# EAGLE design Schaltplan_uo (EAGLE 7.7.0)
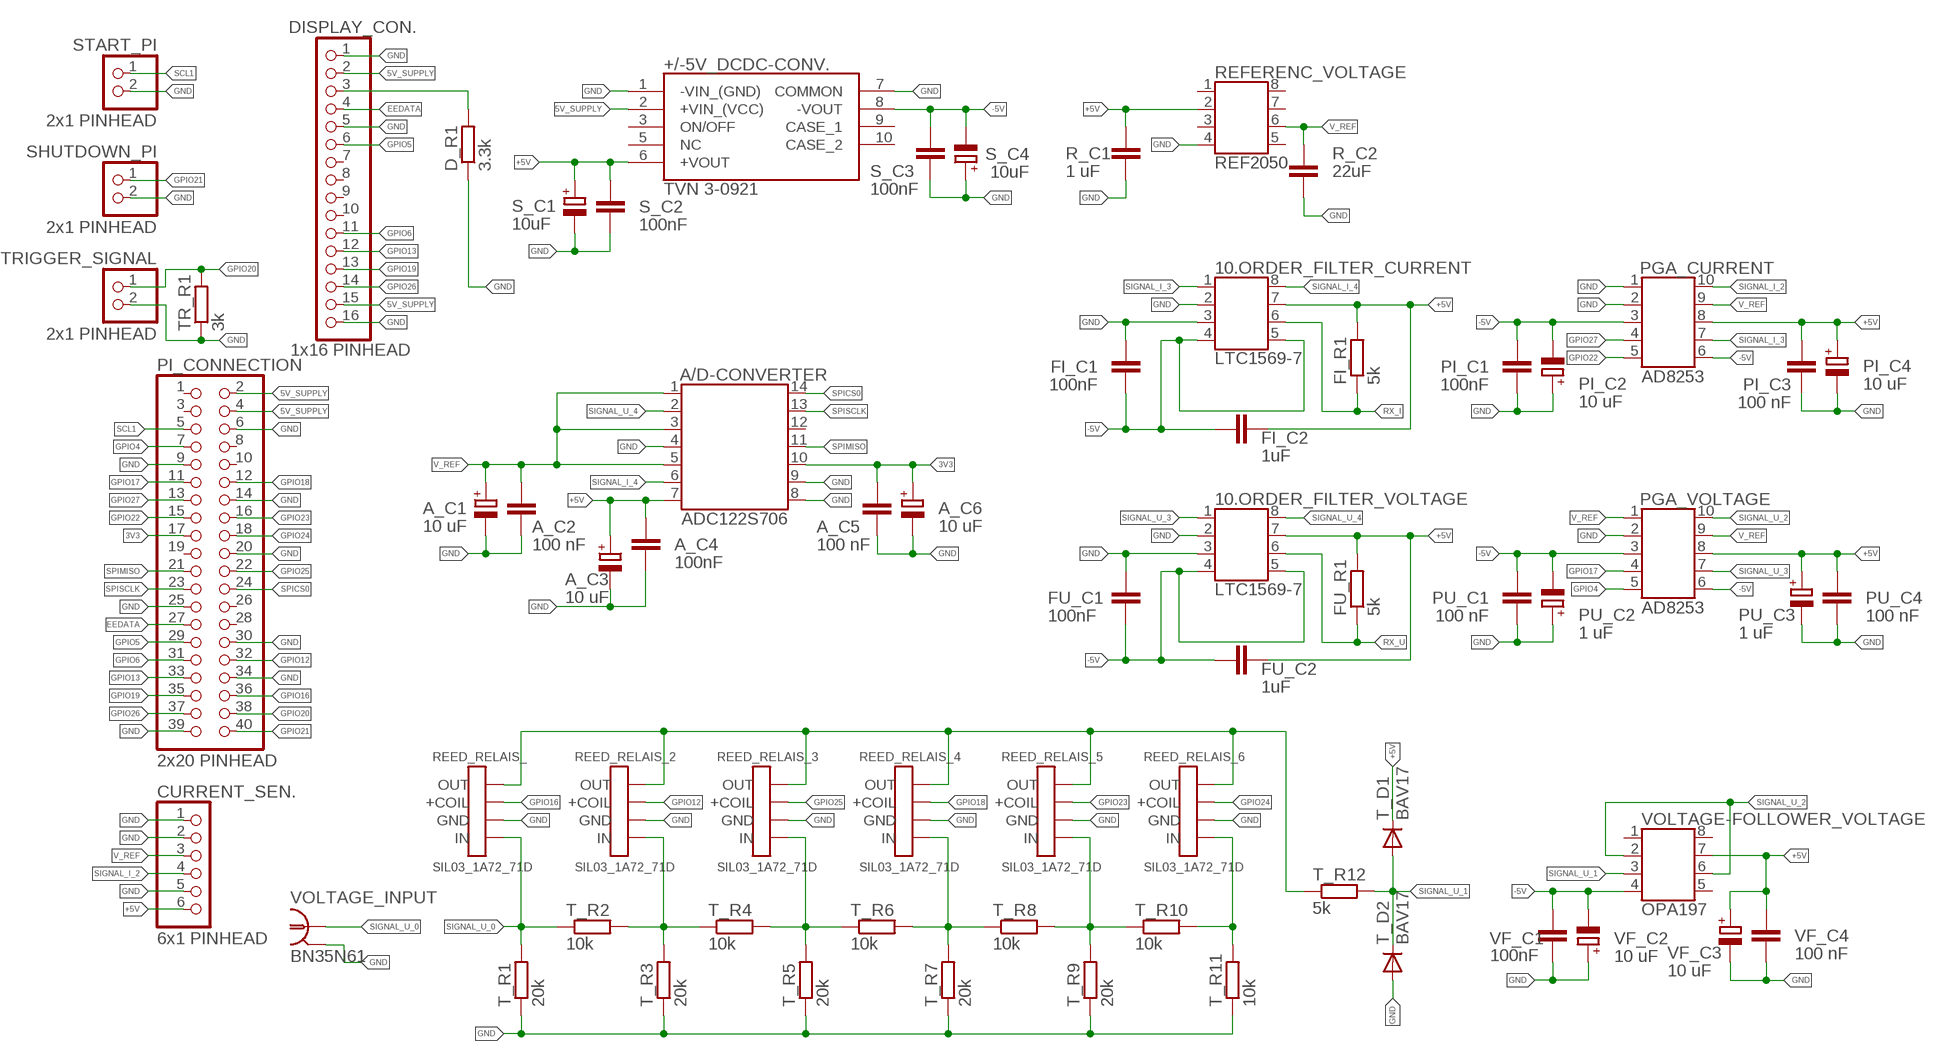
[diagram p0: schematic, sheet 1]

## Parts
10.ORDER_FILTER_CURRENT  LTC1569-7  SSOP8_TO_DIP8  [SSOP8_TO_DIP8]
10.ORDER_FILTER_VOLTAGE  LTC1569-7  SSOP8_TO_DIP8  [SSOP8_TO_DIP8]
+/-5V_DCDC-CONV.  TVN 3-0921  TVN_3-1223  [TVN32419]
A/D-CONVERTER  ADC122S706  SSOP14_TO_DIP14-6  [SSOP14_TO_DIP14-6]
A_C1  10 uF  CPOL-EUE2.5-6  [E2,5-6]
A_C2  100 nF  C-EU025-030X050  [C025-030X050]
A_C3  10 uF  CPOL-EUE2.5-6  [E2,5-6]
A_C4  100nF  C-EU025-030X050  [C025-030X050]
A_C5  100 nF  C-EU025-030X050  [C025-030X050]
A_C6  10 uF  CPOL-EUE2.5-6  [E2,5-6]
CURRENT_SEN.  6x1 PINHEAD  PINHD-1X6  [1X06]
D_R1  3.3k  R-EU_0207/10  [0207/10]
DISPLAY_CON.  1x16 PINHEAD  PINHD-1X16  [1X16]
FI_C1  100nF  C-EU025-030X050  [C025-030X050]
FI_C2  1uF  C-EU025-030X050  [C025-030X050]
FI_R1  5k  R-EU_0207/10  [0207/10]
FU_C1  100nF  C-EU025-030X050  [C025-030X050]
FU_C2  1uF  C-EU025-030X050  [C025-030X050]
FU_R1  5k  R-EU_0207/10  [0207/10]
PGA_CURRENT  AD8253  SSOP10_TO_DIP10  [SSOP10_TO_DIP10]
PGA_VOLTAGE  AD8253  SSOP10_TO_DIP10  [SSOP10_TO_DIP10]
PI_C1  100nF  C-EU025-030X050  [C025-030X050]
PI_C2  10 uF  CPOL-EUE2.5-6  [E2,5-6]
PI_C3  100 nF  C-EU025-030X050  [C025-030X050]
PI_C4  10 uF  CPOL-EUE2.5-6  [E2,5-6]
PI_CONNECTION  2x20 PINHEAD  PINHD-2X20  [2X20]
PU_C1  100 nF  C-EU025-030X050  [C025-030X050]
PU_C2  1 uF  CPOL-EUE2.5-6  [E2,5-6]
PU_C3  1 uF  CPOL-EUE2.5-6  [E2,5-6]
PU_C4  100 nF  C-EU025-030X050  [C025-030X050]
R_C1  1 uF  C-EU025-030X050  [C025-030X050]
R_C2  22uF  C-EU025-030X050  [C025-030X050]
REED_RELAIS_  SIL03_1A72_71D  REED_REALIS_SIL03_1A72_71D  [REED_RELAIS_SIL03_1A72_71D]
REED_RELAIS_2  SIL03_1A72_71D  REED_REALIS_SIL03_1A72_71D  [REED_RELAIS_SIL03_1A72_71D]
REED_RELAIS_3  SIL03_1A72_71D  REED_REALIS_SIL03_1A72_71D  [REED_RELAIS_SIL03_1A72_71D]
REED_RELAIS_4  SIL03_1A72_71D  REED_REALIS_SIL03_1A72_71D  [REED_RELAIS_SIL03_1A72_71D]
REED_RELAIS_5  SIL03_1A72_71D  REED_REALIS_SIL03_1A72_71D  [REED_RELAIS_SIL03_1A72_71D]
REED_RELAIS_6  SIL03_1A72_71D  REED_REALIS_SIL03_1A72_71D  [REED_RELAIS_SIL03_1A72_71D]
REFERENC_VOLTAGE  REF2050  SSOP8_TO_DIP8  [SSOP8_TO_DIP8]
S_C1  10uF  CPOL-EUE2.5-6  [E2,5-6]
S_C2  100nF  C-EU025-030X050  [C025-030X050]
S_C3  100nF  C-EU025-030X050  [C025-030X050]
S_C4  10uF  CPOL-EUE2.5-6  [E2,5-6]
SHUTDOWN_PI  2x1 PINHEAD  PINHD-1X2  [1X02]
START_PI  2x1 PINHEAD  PINHD-1X2  [1X02]
T_D1  BAV17  [DO35-10]
T_D2  BAV17  [DO35-10]
T_R1  20k  R-EU_0207/10  [0207/10]
T_R2  10k  R-EU_0207/10  [0207/10]
T_R3  20k  R-EU_0207/10  [0207/10]
T_R4  10k  R-EU_0207/10  [0207/10]
T_R5  20k  R-EU_0207/10  [0207/10]
T_R6  10k  R-EU_0207/10  [0207/10]
T_R7  20k  R-EU_0207/10  [0207/10]
T_R8  10k  R-EU_0207/10  [0207/10]
T_R9  20k  R-EU_0207/10  [0207/10]
T_R10  10k  R-EU_0207/10  [0207/10]
T_R11  10k  R-EU_0207/10  [0207/10]
T_R12  5k  R-EU_0207/10  [0207/10]
TR_R1  3k  R-EU_0207/10  [0207/10]
TRIGGER_SIGNAL  2x1 PINHEAD  PINHD-1X2  [1X02]
VF_C1  100nF  C-EU025-030X050  [C025-030X050]
VF_C2  10 uF  CPOL-EUE2.5-6  [E2,5-6]
VF_C3  10 uF  CPOL-EUE2.5-6  [E2,5-6]
VF_C4  100 nF  C-EU025-030X050  [C025-030X050]
VOLTAGE-FOLLOWER_VOLTAGE  OPA197  SSOP8_TO_DIP8  [SSOP8_TO_DIP8]
VOLTAGE_INPUT  BN35N61  [B35N61]

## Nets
3V3: A/D-CONVERTER.10 A_C5.1 A_C6.+ PI_CONNECTION.17
5V_SUPPLY: +/-5V_DCDC-CONV..2(+VIN_(VCC)) DISPLAY_CON..2 DISPLAY_CON..15 PI_CONNECTION.2 PI_CONNECTION.4
+5V: 10.ORDER_FILTER_CURRENT.7 10.ORDER_FILTER_VOLTAGE.7 +/-5V_DCDC-CONV..6(+VOUT) A/D-CONVERTER.7 A_C3.+ A_C4.1 CURRENT_SEN..6 FI_C2.2 FI_R1.2 FU_C2.1 FU_R1.2 PGA_CURRENT.8 PGA_VOLTAGE.8 PI_C3.1 PI_C4.+ PU_C3.+ PU_C4.1 R_C1.1 REFERENC_VOLTAGE.2 S_C1.+ S_C2.1 T_D1.C VF_C3.+ VF_C4.1 VOLTAGE-FOLLOWER_VOLTAGE.7
-5V: 10.ORDER_FILTER_CURRENT.4 10.ORDER_FILTER_CURRENT.5 10.ORDER_FILTER_VOLTAGE.4 10.ORDER_FILTER_VOLTAGE.5 +/-5V_DCDC-CONV..8(-VOUT) FI_C1.1 FI_C2.1 FU_C1.1 FU_C2.2 PGA_CURRENT.3 PGA_CURRENT.6 PGA_VOLTAGE.3 PGA_VOLTAGE.6 PI_C1.1 PI_C2.- PU_C1.1 PU_C2.- S_C3.1 S_C4.- VF_C1.1 VF_C2.- VOLTAGE-FOLLOWER_VOLTAGE.4
EEDATA: DISPLAY_CON..4 PI_CONNECTION.27
GND: 10.ORDER_FILTER_CURRENT.2 10.ORDER_FILTER_CURRENT.3 10.ORDER_FILTER_VOLTAGE.2 10.ORDER_FILTER_VOLTAGE.3 +/-5V_DCDC-CONV..1(-VIN_(GND)) +/-5V_DCDC-CONV..7(COMMON) A/D-CONVERTER.4 A/D-CONVERTER.8 A/D-CONVERTER.9 A_C1.- A_C2.2 A_C3.- A_C4.2 A_C5.2 A_C6.- CURRENT_SEN..1 CURRENT_SEN..2 CURRENT_SEN..5 D_R1.1 DISPLAY_CON..1 DISPLAY_CON..5 DISPLAY_CON..16 FI_C1.2 FU_C1.2 PGA_CURRENT.1 PGA_CURRENT.2 PGA_VOLTAGE.2 PI_C1.2 PI_C2.+ PI_C3.2 PI_C4.- PI_CONNECTION.6 PI_CONNECTION.9 PI_CONNECTION.14 PI_CONNECTION.20 PI_CONNECTION.25 PI_CONNECTION.30 PI_CONNECTION.34 PI_CONNECTION.39 PU_C1.2 PU_C2.+ PU_C3.- PU_C4.2 R_C1.2 R_C2.2 REED_RELAIS_2.P$3(GND) REED_RELAIS_3.P$3(GND) REED_RELAIS_4.P$3(GND) REED_RELAIS_5.P$3(GND) REED_RELAIS_6.P$3(GND) REED_RELAIS_.P$3(GND) REFERENC_VOLTAGE.4 S_C1.- S_C2.2 S_C3.2 S_C4.+ SHUTDOWN_PI.2 START_PI.2 T_D2.A T_R1.1 T_R3.1 T_R5.1 T_R7.1 T_R9.1 T_R11.1 TR_R1.1 TRIGGER_SIGNAL.2 VF_C1.2 VF_C2.+ VF_C3.- VF_C4.2 VOLTAGE_INPUT.2 VOLTAGE_INPUT.3 VOLTAGE_INPUT.4 VOLTAGE_INPUT.5
GPIO4: PGA_VOLTAGE.5 PI_CONNECTION.7
GPIO5: DISPLAY_CON..6 PI_CONNECTION.29
GPIO6: DISPLAY_CON..11 PI_CONNECTION.31
GPIO12: PI_CONNECTION.32 REED_RELAIS_2.P$2(+COIL)
GPIO13: DISPLAY_CON..12 PI_CONNECTION.33
GPIO16: PI_CONNECTION.36 REED_RELAIS_.P$2(+COIL)
GPIO17: PGA_VOLTAGE.4 PI_CONNECTION.11
GPIO18: PI_CONNECTION.12 REED_RELAIS_4.P$2(+COIL)
GPIO19: DISPLAY_CON..13 PI_CONNECTION.35
GPIO20: PI_CONNECTION.38 TR_R1.2 TRIGGER_SIGNAL.1
GPIO21: PI_CONNECTION.40 SHUTDOWN_PI.1
GPIO22: PGA_CURRENT.5 PI_CONNECTION.15
GPIO23: PI_CONNECTION.16 REED_RELAIS_5.P$2(+COIL)
GPIO24: PI_CONNECTION.18 REED_RELAIS_6.P$2(+COIL)
GPIO25: PI_CONNECTION.22 REED_RELAIS_3.P$2(+COIL)
GPIO26: DISPLAY_CON..14 PI_CONNECTION.37
GPIO27: PGA_CURRENT.4 PI_CONNECTION.13
N$2: REED_RELAIS_2.P$1(OUT) REED_RELAIS_3.P$1(OUT) REED_RELAIS_4.P$1(OUT) REED_RELAIS_5.P$1(OUT) REED_RELAIS_6.P$1(OUT) REED_RELAIS_.P$1(OUT) T_R12.1
N$3: D_R1.2 DISPLAY_CON..3
N$42: REED_RELAIS_2.P$4(IN) T_R2.2 T_R3.2 T_R4.1
N$43: REED_RELAIS_3.P$4(IN) T_R4.2 T_R5.2 T_R6.1
N$44: REED_RELAIS_4.P$4(IN) T_R6.2 T_R7.2 T_R8.1
N$45: REED_RELAIS_5.P$4(IN) T_R8.2 T_R9.2 T_R10.1
N$46: REED_RELAIS_6.P$4(IN) T_R10.2 T_R11.2
RX_I: 10.ORDER_FILTER_CURRENT.6 FI_R1.1
RX_U: 10.ORDER_FILTER_VOLTAGE.6 FU_R1.1
SCL1: PI_CONNECTION.5 START_PI.1
SIGNAL_I_2: CURRENT_SEN..4 PGA_CURRENT.10
SIGNAL_I_3: 10.ORDER_FILTER_CURRENT.1 PGA_CURRENT.7
SIGNAL_I_4: 10.ORDER_FILTER_CURRENT.8 A/D-CONVERTER.6
SIGNAL_U_0: REED_RELAIS_.P$4(IN) T_R1.2 T_R2.1 VOLTAGE_INPUT.1
SIGNAL_U_1: T_D1.A T_D2.C T_R12.2 VOLTAGE-FOLLOWER_VOLTAGE.3
SIGNAL_U_2: PGA_VOLTAGE.10 VOLTAGE-FOLLOWER_VOLTAGE.2 VOLTAGE-FOLLOWER_VOLTAGE.6
SIGNAL_U_3: 10.ORDER_FILTER_VOLTAGE.1 PGA_VOLTAGE.7
SIGNAL_U_4: 10.ORDER_FILTER_VOLTAGE.8 A/D-CONVERTER.2
SPICS0: A/D-CONVERTER.14 PI_CONNECTION.24
SPIMISO: A/D-CONVERTER.11 PI_CONNECTION.21
SPISCLK: A/D-CONVERTER.13 PI_CONNECTION.23
V_REF: A/D-CONVERTER.1 A/D-CONVERTER.3 A/D-CONVERTER.5 A_C1.+ A_C2.1 CURRENT_SEN..3 PGA_CURRENT.9 PGA_VOLTAGE.1 PGA_VOLTAGE.9 R_C2.1 REFERENC_VOLTAGE.6
Unconnected: +/-5V_DCDC-CONV..3(ON/OFF) +/-5V_DCDC-CONV..5(NC) +/-5V_DCDC-CONV..9(CASE_1) +/-5V_DCDC-CONV..10(CASE_2) A/D-CONVERTER.12 DISPLAY_CON..7 DISPLAY_CON..8 DISPLAY_CON..9 DISPLAY_CON..10 PI_CONNECTION.1 PI_CONNECTION.3 PI_CONNECTION.8 PI_CONNECTION.10 PI_CONNECTION.19 PI_CONNECTION.26 PI_CONNECTION.28 REFERENC_VOLTAGE.1 REFERENC_VOLTAGE.3 REFERENC_VOLTAGE.5 REFERENC_VOLTAGE.7 REFERENC_VOLTAGE.8 VOLTAGE-FOLLOWER_VOLTAGE.1 VOLTAGE-FOLLOWER_VOLTAGE.5 VOLTAGE-FOLLOWER_VOLTAGE.8

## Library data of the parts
10.ORDER_FILTER_CURRENT 10.ORDER_FILTER_VOLTAGE REFERENC_VOLTAGE VOLTAGE-FOLLOWER_VOLTAGE = OWN_Library:SSOP8_TO_DIP8
+/-5V_DCDC-CONV. = TVN_3-1223:TVN_3-1223: Isolated DC/DC Converters 3W 9-18Vin SIP-8 +/-15Vout +/-100mA Source: Datasheet; ALLIED_NUMBER: 71099550; ALLIED_PRICE-STOCK: https://www.alliedelec.com/traco-power-tvn-3-1223/71099550/; DESCRIPTION: Isolated DC/DC Converters 3W 9-18Vin SIP-8 +/-15Vout +/-100mA; HEIGHT: 11mm; MANUFACTURER_NAME: Traco Power; MANUFACTURER_PART_NUMBER: TVN 3-1223; MOUSER_PART_NUMBER: 495-TVN3-1223; MOUSER_PRICE-STOCK: https://www.mouser.com/Search/Refine.aspx?Keyword=495-TVN3-1223; RS_PART_NUMBER: 1466094; RS_PRICE-STOCK: https://uk.rs-online.com/web/p/products/1466094
A/D-CONVERTER = OWN_Library:SSOP14_TO_DIP14-6: SSOP14 SMD to DIP14-6 ADAPTER
A_C1 A_C3 A_C6 PI_C2 PI_C4 PU_C2 PU_C3 S_C1 S_C4 VF_C2 VF_C3 = rcl:CPOL-EU: POLARIZED CAPACITOR, European symbol
A_C2 A_C4 A_C5 FI_C1 FI_C2 FU_C1 FU_C2 PI_C1 PI_C3 PU_C1 PU_C4 R_C1 R_C2 S_C2 S_C3 VF_C1 VF_C4 = rcl:C-EU: CAPACITOR, European symbol
CURRENT_SEN. = pinhead:PINHD-1X6: PIN HEADER
D_R1 FI_R1 FU_R1 T_R1-T_R12 TR_R1 = rcl:R-EU_: RESISTOR, European symbol
DISPLAY_CON. = pinhead:PINHD-1X16: PIN HEADER
PGA_CURRENT PGA_VOLTAGE = OWN_Library:SSOP10_TO_DIP10
PI_CONNECTION = pinhead:PINHD-2X20: PIN HEADER
REED_RELAIS_ REED_RELAIS_2-REED_RELAIS_6 = OWN_Library:REED_REALIS_SIL03_1A72_71D
SHUTDOWN_PI START_PI TRIGGER_SIGNAL = pinhead:PINHD-1X2: PIN HEADER
T_D1 T_D2 = diode:BAV17: DIODE
VOLTAGE_INPUT = con-coax:BN35N61: BNC CONNECTOR; OC_FARNELL: unknown; OC_NEWARK: unknown

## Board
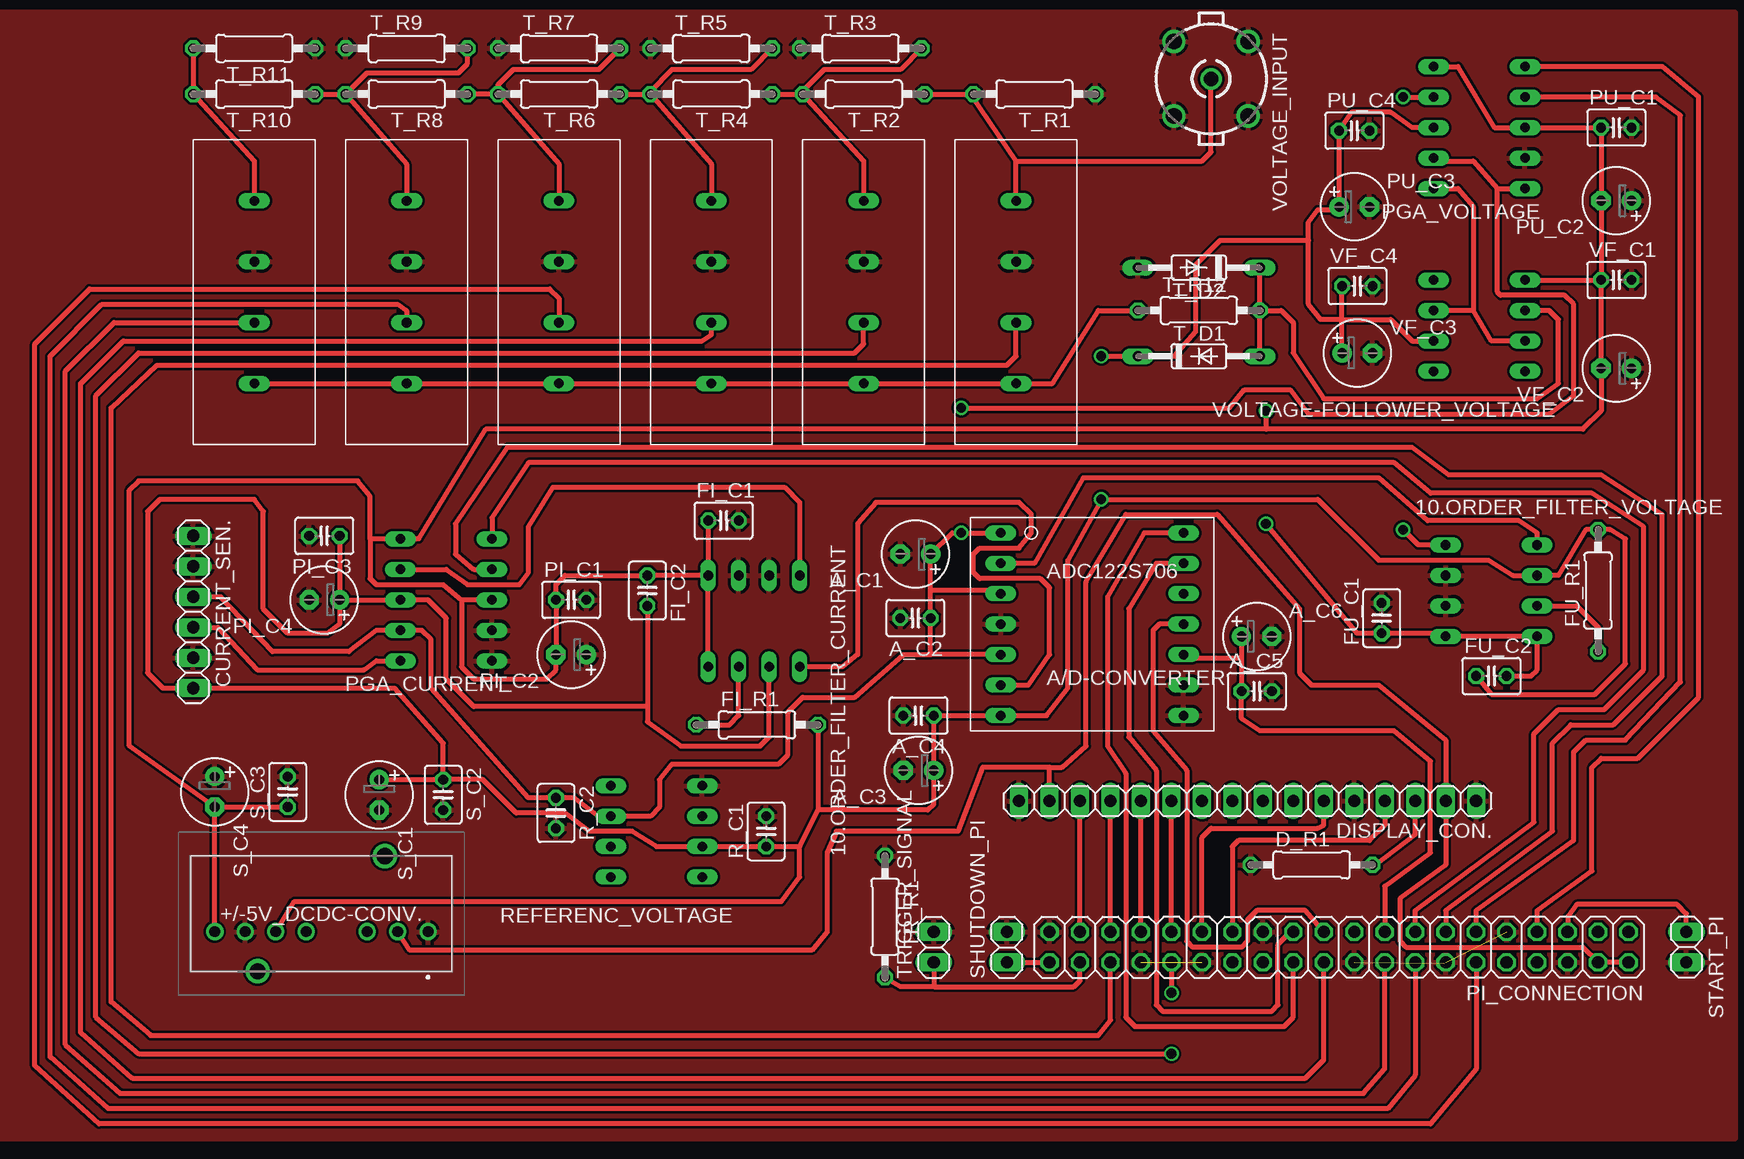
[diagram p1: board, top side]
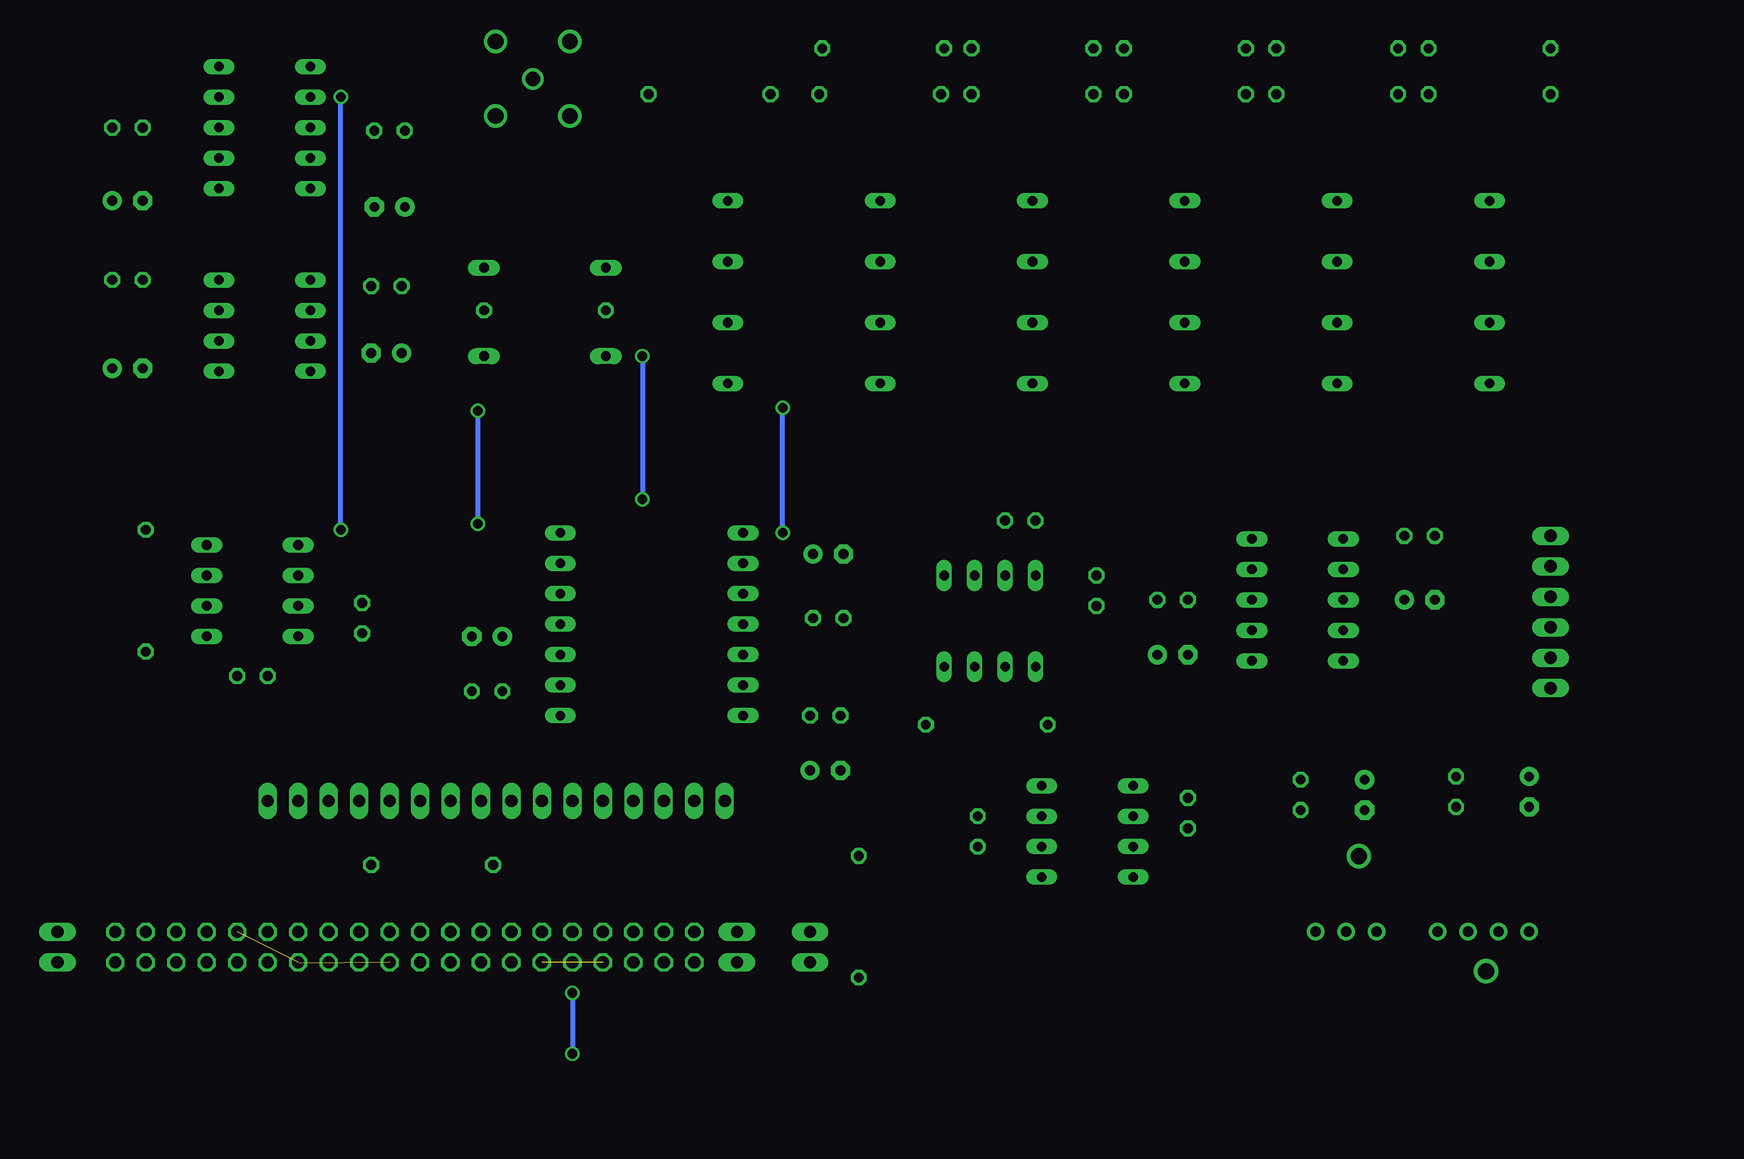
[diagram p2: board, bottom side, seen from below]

No outline drawn. Coordinates in mm, seen from the top.
Copper layers (1*16): Top 0.035mm / dielectric 1.5mm / Bottom 0.035mm
Design rules "default": minimum track width 10mil, minimum drill 24mil, track to track 8mil, track to pad 8mil, pad to pad 8mil, via to via 8mil, smd to smd 8mil, copper to edge 40mil, drill to drill 8mil, minimum pad ring 10mil, minimum via ring 8mil, stop-mask expansion 4mil, vias tented up to drill 0mil, thermal gap 10mil

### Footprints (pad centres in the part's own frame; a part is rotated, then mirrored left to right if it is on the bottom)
SSOP8_TO_DIP8 = drill 0.8 long: 1 -5.08,2.54; 2 -5.08,0; 3 -5.08,-2.54; 4 -5.08,-5.08; 5 2.54,-5.08; 6 2.54,-2.54; 7 2.54,0; 8 2.54,2.54
TVN32419 = drill 0.89 pad 1.446: 1 -8.9,1.5; 2 -6.36,1.5; 3 -3.82,1.5; 5 1.26,1.5; 6 3.8,1.5; 7 6.34,1.5; 8 8.88,1.5 | drill 1.35 pad 2.025: 9 -5.3,-4.8; 10 5.3,4.8
SSOP14_TO_DIP14-6 = drill 0.8 long: 1 -7.62,7.62; 2 -7.62,5.08; 3 -7.62,2.54; 4 -7.62,0; 5 -7.62,-2.54; 6 -7.62,-5.08; 7 -7.62,-7.62; 8 7.62,-7.62; 9 7.62,-5.08; 10 7.62,-2.54; 11 7.62,0; 12 7.62,2.54; 13 7.62,5.08; 14 7.62,7.62
E2,5-6 = drill 0.813 pad 1.6: + -1.27,0 | drill 0.813 pad 1.6 octagon: - 1.27,0
C025-030X050 = drill 0.813 octagon: 1 -1.27,0; 2 1.27,0
1X06 = drill 1.016 long: 1 -6.35,0; 2 -3.81,0; 3 -1.27,0; 4 1.27,0; 5 3.81,0; 6 6.35,0
0207/10 = drill 0.813 octagon: 1 -5.08,0; 2 5.08,0
1X16 = drill 1.016 long: 1 -19.05,0; 2 -16.51,0; 3 -13.97,0; 4 -11.43,0; 5 -8.89,0; 6 -6.35,0; 7 -3.81,0; 8 -1.27,0; 9 1.27,0; 10 3.81,0; 11 6.35,0; 12 8.89,0; 13 11.43,0; 14 13.97,0; 15 16.51,0; 16 19.05,0
SSOP10_TO_DIP10 = drill 0.8 long: 1 -2.54,2.54; 2 -2.54,0; 3 -2.54,-2.54; 4 -2.54,-5.08; 5 -2.54,-7.62; 6 5.08,-7.62; 7 5.08,-5.08; 8 5.08,-2.54; 9 5.08,0; 10 5.08,2.54
2X20 = drill 1.016 octagon: 1 -24.13,-1.27; 2 -24.13,1.27; 3 -21.59,-1.27; 4 -21.59,1.27; 5 -19.05,-1.27; 6 -19.05,1.27; 7 -16.51,-1.27; 8 -16.51,1.27; 9 -13.97,-1.27; 10 -13.97,1.27; 11 -11.43,-1.27; 12 -11.43,1.27; 13 -8.89,-1.27; 14 -8.89,1.27; 15 -6.35,-1.27; 16 -6.35,1.27; 17 -3.81,-1.27; 18 -3.81,1.27; 19 -1.27,-1.27; 20 -1.27,1.27; 21 1.27,-1.27; 22 1.27,1.27; 23 3.81,-1.27; 24 3.81,1.27; 25 6.35,-1.27; 26 6.35,1.27; 27 8.89,-1.27; 28 8.89,1.27; 29 11.43,-1.27; 30 11.43,1.27; 31 13.97,-1.27; 32 13.97,1.27; 33 16.51,-1.27; 34 16.51,1.27; 35 19.05,-1.27; 36 19.05,1.27; 37 21.59,-1.27; 38 21.59,1.27; 39 24.13,-1.27; 40 24.13,1.27
REED_RELAIS_SIL03_1A72_71D = drill 0.8 long: P$1 0,0; P$2 0,-5.08; P$3 0,-10.16; P$4 0,-15.24
1X02 = drill 1.016 long: 1 -1.27,0; 2 1.27,0
DO35-10 = drill 0.813 long: A 5.08,0; C -5.08,0
B35N61 = drill 1.2: 1 0,0 | drill 1.3: 2 3.099,3.099; 3 -3.099,3.099; 4 -3.099,-3.099; 5 3.099,-3.099

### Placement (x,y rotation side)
10.ORDER_FILTER_CURRENT  64.26,41.91 270 top
10.ORDER_FILTER_VOLTAGE  125.73,46.99 0 top
+/-5V_DCDC-CONV.  26.92,18.8 180 top
A/D-CONVERTER  91.19,42.93 0 top
A_C1  76.45,48.77 180 top
A_C2  76.45,43.43 180 top
A_C3  76.71,30.73 180 top
A_C4  76.71,35.31 180 top
A_C5  104.9,37.34 0 top
A_C6  104.9,41.91 0 top
CURRENT_SEN.  16.26,43.94 270 top
D_R1  109.47,22.86 0 top
DISPLAY_CON.  104.14,28.19 180 top
FI_C1  60.45,51.56 0 top
FI_C2  54.1,45.72 270 top
FI_R1  63.25,34.54 0 top
FU_C1  115.32,43.43 90 top
FU_C2  124.46,38.61 0 top
FU_R1  133.35,45.72 90 top
PGA_CURRENT  38.61,42.42 180 top
PGA_VOLTAGE  124.71,81.79 180 top
PI_C1  47.75,44.96 0 top
PI_C2  47.75,40.39 180 top
PI_C3  27.18,50.29 180 top
PI_C4  27.18,44.96 180 top
PI_CONNECTION  111.76,16 180 top
PU_C1  134.87,84.33 0 top
PU_C2  134.87,78.23 180 top
PU_C3  113.03,77.72 0 top
PU_C4  113.03,84.07 0 top
R_C1  64.01,25.65 90 top
R_C2  46.48,27.18 270 top
REED_RELAIS_  84.84,62.99 180 top
REED_RELAIS_2  72.14,62.99 180 top
REED_RELAIS_3  59.44,62.99 180 top
REED_RELAIS_4  46.74,62.99 180 top
REED_RELAIS_5  34.04,62.99 180 top
REED_RELAIS_6  21.34,62.99 180 top
REFERENC_VOLTAGE  53.59,24.38 180 top
S_C1  31.75,28.7 270 top
S_C2  37.08,28.7 270 top
S_C3  24.13,28.96 90 top
S_C4  18.03,28.96 270 top
SHUTDOWN_PI  84.07,16 90 top
START_PI  140.72,16 270 top
T_D1  100.08,65.28 0 top
T_D2  100.08,72.64 180 top
T_R1  86.36,87.12 180 top
T_R2  72.14,87.12 180 top
T_R3  71.88,90.93 0 top
T_R4  59.44,87.12 180 top
T_R5  59.44,90.93 0 top
T_R6  46.74,87.12 180 top
T_R7  46.74,90.93 0 top
T_R8  34.04,87.12 180 top
T_R9  34.04,90.93 0 top
T_R10  21.34,87.12 180 top
T_R11  21.34,90.93 180 top
T_R12  100.08,69.09 0 top
TR_R1  73.91,18.54 270 top
TRIGGER_SIGNAL  77.98,16 90 top
VF_C1  134.87,71.63 0 top
VF_C2  134.87,64.26 180 top
VF_C3  113.28,65.53 0 top
VF_C4  113.28,71.12 0 top
VOLTAGE-FOLLOWER_VOLTAGE  122.17,66.55 180 top
VOLTAGE_INPUT  101.09,88.39 270 top

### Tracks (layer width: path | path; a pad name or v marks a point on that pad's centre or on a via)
3V3
  Top 0.406: PI_CONNECTION.17 115.57,21.08 119.38,23.88 119.38,31.5 116.33,34.04 105.16,34.04 103.63,35.05 A_C5.1 103.63,40.13 | A_C6.+ 103.63,40.13 | A/D-CONVERTER.10 99.06,40.13 103.63,40.13
5V_SUPPLY
  Top 0.406: 87.63,30.99 82.04,30.99 80.01,25.65 69.85,25.65 69.09,23.88 69.09,17.27 67.82,15.75 34.29,15.75 33.3,17.3 +/-5V_DCDC-CONV..2 | PI_CONNECTION.2 PI_CONNECTION.4 132.08,16 117.35,16 116.84,16.51 116.84,20.07 120.65,22.86 DISPLAY_CON..2 120.65,33.27 115.06,37.85 109.47,37.85 108.46,38.86 108.46,44.2 101.6,52.07 93.98,52.07 90.68,46.48 90.68,32.77 88.65,30.99 87.63,30.99 | DISPLAY_CON..15 87.63,30.99
+5V  (via drill 0.8)
  Top 0.406: FU_C2.1 124.46,37.08 133.1,37.08 135.64,39.62 135.64,50.04 134.37,50.8 FU_R1.2 132.33,50.8 130.05,46.99 10.ORDER_FILTER_VOLTAGE.7 126.24,46.99 124.21,48.26 115.06,48.26 109.98,53.34 v91.95,53.34 89.15,48.26 89.15,37.59 87.38,35.31 A/D-CONVERTER.7 A_C4.1 A_C3.+ 77.98,27.94 77.47,27.43 68.33,27.43 | PI_C4.+ 28.45,42.93 27.43,42.16 24.13,42.16 22.1,44.2 22.1,52.32 21.34,53.34 13.46,53.34 12.45,52.32 12.45,38.86 13.72,37.59 CURRENT_SEN..6 33.02,37.59 37.08,33.02 S_C2.1 | S_C1.+ S_C2.1 | PI_C3.1 PI_C4.+ | PI_C4.+ PGA_CURRENT.8 35.81,44.96 37.34,43.43 37.34,38.35 39.62,36.07 54.1,36.07 | S_C2.1 40.39,29.97 43.18,27.18 47.24,27.18 49.28,25.65 52.83,25.65 54.86,24.38 REFERENC_VOLTAGE.2 R_C1.1 66.8,24.38 | FI_R1.2 68.33,27.43 | +/-5V_DCDC-CONV..6 24.67,19.81 65.28,19.81 66.8,21.84 66.8,24.38 | 68.33,27.43 66.8,24.38 | v91.95,65.28 T_D1.C 98.04,65.28 99.82,67.31 99.82,72.9 101.85,74.93 109.22,74.93 | 112.01,68.33 VF_C4.1 | 112.01,68.33 116.08,68.33 117.86,66.55 VOLTAGE-FOLLOWER_VOLTAGE.7 | VF_C3.+ 112.01,68.33 | 112.01,68.33 110.24,68.33 109.22,69.6 109.22,74.93 | PGA_VOLTAGE.8 117.86,84.33 116.08,85.6 112.78,85.6 PU_C4.1 PU_C3.+ 111.51,77.47 109.98,77.47 109.22,76.45 109.22,74.93 | FI_C2.2 54.1,36.07 | 54.1,36.07 54.1,34.8 56.9,32.77 63.5,32.77 64.26,33.53 10.ORDER_FILTER_CURRENT.7
  Bottom 0.406: v91.95,65.28 v91.95,53.34
-5V  (via drill 0.8)
  Top 0.406: FU_C2.2 127.76,38.61 128.27,39.12 10.ORDER_FILTER_VOLTAGE.5 10.ORDER_FILTER_VOLTAGE.4 120.4,42.16 FU_C1.1 113.28,42.16 v105.66,51.31 | 10.ORDER_FILTER_CURRENT.4 FI_C2.1 47.24,46.99 46.48,46.23 PI_C1.1 PI_C2.- 46.48,39.12 45.72,38.35 39.62,38.35 38.61,39.37 38.61,44.96 | 18.05,27.69 18.04,27.68 S_C4.- +/-5V_DCDC-CONV..8 | 18.05,27.69 S_C3.1 | PGA_CURRENT.3 38.61,44.96 | 18.05,27.69 10.92,32.79 10.92,54.1 11.68,54.86 29.97,54.86 30.99,53.59 30.99,50.04 | PGA_CURRENT.6 31.75,50.04 | PGA_CURRENT.6 30.99,50.04 | 30.99,50.04 30.99,46.74 31.5,46.23 37.08,46.23 38.61,44.96 | 105.66,59.18 40.64,59.18 35.05,50.04 PGA_CURRENT.6 | v105.66,60.71 105.66,59.18 | PGA_VOLTAGE.6 121.67,89.41 124.71,84.33 PGA_VOLTAGE.3 PU_C1.1 PU_C2.- VF_C1.1 | VF_C1.1 VF_C2.- 133.6,60.71 132.08,59.18 105.66,59.18 | VOLTAGE-FOLLOWER_VOLTAGE.4 VF_C1.1 | 10.ORDER_FILTER_CURRENT.5 10.ORDER_FILTER_CURRENT.4 | FI_C1.1 10.ORDER_FILTER_CURRENT.4
  Bottom 0.406: v105.66,51.31 v105.66,60.71
EEDATA
  Top 0.406: DISPLAY_CON..4 115.57,26.16 114.3,24.89 103.38,24.89 102.87,24.38 PI_CONNECTION.27
GND  (3 unrouted)
  Top 0.254: 120.52,14.67 PI_CONNECTION.14
  pour Top: 0,93.98 144.78,93.98 144.78,0 0,0
GPIO4
  Top 0.406: PI_CONNECTION.7 128.27,19.05 132.84,22.35 132.84,30.99 133.6,31.75 136.65,31.75 141.73,36.83 141.73,86.87 138.68,89.41 PGA_VOLTAGE.5
GPIO5
  Top 0.406: PI_CONNECTION.29 100.33,25.15 101.09,25.91 109.98,25.91 110.49,26.16 DISPLAY_CON..6
GPIO6
  Top 0.406: PI_CONNECTION.31 DISPLAY_CON..11
GPIO12  (via drill 0.8)
  Top 0.406: v97.79,7.11 11.68,7.11 8.13,10.16 8.13,61.98 11.68,65.53 71.37,65.53 72.14,66.29 REED_RELAIS_2.P$2 | PI_CONNECTION.32 v97.79,12.19
  Bottom 0.406: v97.79,12.19 v97.79,7.11
GPIO13
  Top 0.406: PI_CONNECTION.33 DISPLAY_CON..12
GPIO16
  Top 0.406: PI_CONNECTION.36 92.71,9.91 91.69,8.64 12.7,8.64 9.4,11.43 9.4,60.96 13.21,64.52 84.07,64.52 84.84,65.28 REED_RELAIS_.P$2
GPIO17
  Top 0.406: PGA_VOLTAGE.4 138.18,86.87 140.21,85.34 140.21,38.1 135.64,33.27 132.33,33.27 131.32,32.26 131.32,24.89 123.19,19.05 PI_CONNECTION.11
GPIO18
  Top 0.406: PI_CONNECTION.12 123.19,5.84 119.38,1.27 8.38,1.27 3.05,6.1 3.05,66.29 7.62,70.87 45.97,70.87 46.74,70.1 REED_RELAIS_4.P$2
GPIO19
  Top 0.406: PI_CONNECTION.35 DISPLAY_CON..13
GPIO20
  Top 0.406: 77.98,12.7 89.66,12.7 90.17,13.21 PI_CONNECTION.38 | TRIGGER_SIGNAL.1 77.98,12.7 | 77.98,12.7 75.18,12.7 TR_R1.2
GPIO21
  Top 0.406: SHUTDOWN_PI.1 PI_CONNECTION.40
GPIO22
  Top 0.406: PGA_CURRENT.5 41.15,51.82 44.2,56.39 116.33,56.39 119.38,53.85 132.84,53.85 137.16,51.05 137.16,39.12 133.86,35.81 130.05,35.81 128.02,33.78 128.02,26.42 118.11,19.05 PI_CONNECTION.15
GPIO23
  Top 0.406: PI_CONNECTION.16 118.11,5.33 115.82,2.54 9.14,2.54 4.32,6.86 4.32,65.28 8.64,69.6 33.27,69.6 34.04,69.09 REED_RELAIS_5.P$2
GPIO24
  Top 0.406: PI_CONNECTION.18 115.57,5.84 113.79,3.81 10.16,3.81 5.59,7.87 5.59,64.01 9.65,68.07 REED_RELAIS_6.P$2
GPIO25
  Top 0.406: PI_CONNECTION.22 110.74,14.48 110.49,14.22 110.49,6.6 108.97,5.08 11.18,5.08 6.86,8.89 6.86,62.99 10.41,66.55 58.67,66.55 59.44,67.06 REED_RELAIS_3.P$2
GPIO26
  Top 0.406: PI_CONNECTION.37 DISPLAY_CON..14
GPIO27
  Top 0.406: PGA_CURRENT.4 39.62,47.5 38.1,48.77 38.1,51.31 42.42,57.66 117.86,57.66 120.9,55.37 133.6,55.37 138.68,52.07 138.68,38.61 134.62,34.54 131.06,34.54 129.54,33.02 129.54,25.65 120.65,19.05 PI_CONNECTION.13
N$2
  Top 0.406: REED_RELAIS_6.P$1 REED_RELAIS_5.P$1 REED_RELAIS_4.P$1 REED_RELAIS_3.P$1 REED_RELAIS_2.P$1 REED_RELAIS_.P$1 87.88,62.99 91.69,69.09 T_R12.1
N$3
  Top 0.406: D_R1.2 114.81,22.86 118.11,25.4 DISPLAY_CON..3
N$42
  Top 0.406: T_R4.1 T_R2.2 | T_R3.2 75.18,89.15 68.83,89.15 67.06,87.38 T_R2.2 | T_R2.2 72.14,81.53 REED_RELAIS_2.P$4
N$43
  Top 0.406: T_R5.2 62.74,89.15 56.13,89.15 54.36,87.38 T_R4.2 | T_R6.1 T_R4.2 | T_R4.2 59.44,81.28 REED_RELAIS_3.P$4
N$44
  Top 0.406: T_R6.2 T_R8.1 | T_R6.2 46.74,81.28 REED_RELAIS_4.P$4 | T_R7.2 50.04,89.15 42.93,89.15 41.66,87.88 T_R6.2
N$45
  Top 0.406: T_R10.1 T_R8.2 | T_R8.2 30.73,88.9 38.35,88.9 39.12,89.66 T_R9.2 | T_R8.2 34.04,81.28 REED_RELAIS_5.P$4
N$46
  Top 0.406: T_R11.2 T_R10.2 21.34,81.53 REED_RELAIS_6.P$4
RX_I
  Top 0.406: FI_R1.1 60.96,34.54 61.72,35.31 10.ORDER_FILTER_CURRENT.6
RX_U
  Top 0.406: 10.ORDER_FILTER_VOLTAGE.6 131.57,44.45 133.35,42.67 FU_R1.1
SCL1
  Top 0.406: START_PI.1 140.72,18.8 139.95,19.56 131.57,19.56 130.81,18.54 PI_CONNECTION.5
SIGNAL_I_2
  Top 0.406: CURRENT_SEN..4 18.29,42.67 21.59,39.12 30.48,39.12 31.5,39.88 PGA_CURRENT.10
SIGNAL_I_3
  Top 0.406: PGA_CURRENT.7 37.34,47.5 39.12,46.23 43.43,46.23 44.2,47.24 44.2,51.05 46.23,54.36 65.53,54.36 66.8,53.09 10.ORDER_FILTER_CURRENT.1
SIGNAL_I_4
  Top 0.406: A/D-CONVERTER.6 85.85,37.85 87.63,40.39 87.63,45.97 86.87,46.74 81.79,46.74 81.28,47.24 81.28,48.77 81.79,49.28 85.09,49.28 86.11,50.55 86.11,52.07 85.09,53.09 73.15,53.09 71.63,51.31 71.63,40.39 70.36,39.37 10.ORDER_FILTER_CURRENT.8
SIGNAL_U_0
  Top 0.406: T_R1.2 81.03,87.12 | T_R2.1 81.03,87.12 | 81.03,87.12 84.84,81.53 | REED_RELAIS_.P$4 84.84,81.53 | 84.84,81.53 100.33,81.53 101.09,82.3 VOLTAGE_INPUT.1
SIGNAL_U_1
  Top 0.406: T_D1.A T_R12.2 | T_R12.2 T_D2.C | T_R12.2 106.93,69.09 107.95,68.07 107.95,65.53 110.49,61.72 128.27,61.72 130.05,62.99 130.05,68.33 129.29,69.09 VOLTAGE-FOLLOWER_VOLTAGE.3
SIGNAL_U_2
  Top 0.406: VOLTAGE-FOLLOWER_VOLTAGE.2 124.46,66.55 122.94,69.09 | 122.94,69.09 VOLTAGE-FOLLOWER_VOLTAGE.6 | PGA_VOLTAGE.10 121.67,79.25 122.94,77.72 122.94,69.09
SIGNAL_U_3  (via drill 0.8)
  Top 0.406: 10.ORDER_FILTER_VOLTAGE.1 118.36,49.53 v117.09,50.8 | v117.09,86.87 PGA_VOLTAGE.7
  Bottom 0.406: v117.09,50.8 v117.09,86.87
SIGNAL_U_4
  Top 0.406: 10.ORDER_FILTER_VOLTAGE.8 128.27,50.55 126.75,51.56 119.13,51.56 115.06,55.12 90.42,55.12 86.36,48.01 A/D-CONVERTER.2
SPICS0
  Top 0.406: A/D-CONVERTER.14 95.5,50.55 92.46,45.21 92.46,32.77 93.98,30.48 93.98,10.16 94.74,9.4 107.19,9.4 107.95,10.16 PI_CONNECTION.24
SPIMISO
  Top 0.406: A/D-CONVERTER.11 96.77,42.93 96.27,42.42 96.27,34.04 99.06,30.73 99.06,16.51 99.57,16 103.63,16 104.14,16.51 104.14,18.29 104.9,19.05 108.97,19.05 PI_CONNECTION.21
SPISCLK
  Top 0.406: A/D-CONVERTER.13 96.52,48.01 94.23,44.2 94.23,33.53 96.52,30.73 96.52,11.18 97.03,10.67 106.17,10.67 106.68,11.18 106.68,16.26 107.7,17.27 PI_CONNECTION.23
V_REF  (via drill 0.8)
  Top 0.406: CURRENT_SEN..3 18.54,45.21 22.86,40.64 29.21,40.64 31.5,42.42 PGA_CURRENT.9 35.31,42.42 36.07,41.66 36.07,37.59 44.2,28.45 R_C2.1 48.01,28.45 50.04,26.92 REFERENC_VOLTAGE.6 54.36,26.92 55.12,27.69 55.12,29.97 56.13,31.24 65.02,31.24 65.79,32 65.79,35.56 67.06,36.83 71.37,36.83 75.44,40.39 77.72,40.39 | PGA_VOLTAGE.9 119.89,81.53 122.94,81.53 124.97,79.25 | 124.97,79.25 PGA_VOLTAGE.1 | v80.26,60.96 102.62,60.96 103.89,62.48 107.7,62.48 109.22,60.45 129.29,60.45 131.32,61.98 131.32,69.6 130.56,70.36 125.22,70.36 124.97,70.61 124.97,79.25 | 77.72,45.72 A_C2.1 77.72,40.39 | 77.72,45.72 A_C1.+ 79.5,50.55 v80.26,50.55 A/D-CONVERTER.1 | A/D-CONVERTER.3 83.31,45.72 77.72,45.72 | A/D-CONVERTER.5 77.72,40.39
  Bottom 0.406: v80.26,50.55 v80.26,60.96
